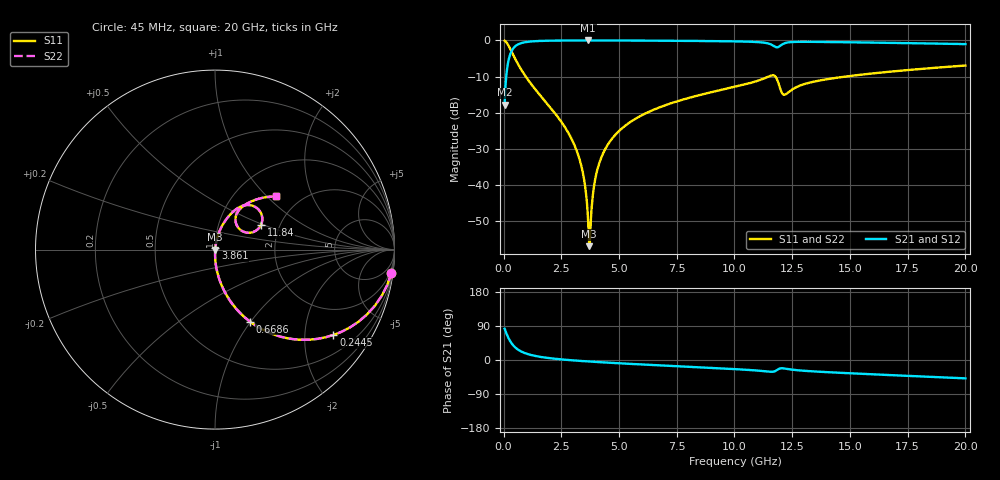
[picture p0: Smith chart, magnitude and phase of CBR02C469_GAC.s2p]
! S-parameter model data by Modelithics Inc.  support@modelithics.com 813-866-6335  Tampa FL USA
! S-Parameter data specifications:
! Substrate: 20-mil Rogers 4350B, substrate thickness, H=0.508mm, Dielectric constant, Er=3.75
! PCB Mounting Pad Footprint: Pad width, PadW=0.32mm , Pad length, PadL=0.37mm , Pad gap, PadG (edge-to-edge)=0.19mm , Reference planes=0.93mm apart
#  GHz  S  MA  R 50
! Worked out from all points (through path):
!   801 points, 45 MHz to 20 GHz, reference 50 ohm
!   highest |S21| = -0.01 dB at 3.662 GHz (marker M1); lowest = -17.7 dB at 45 MHz (marker M2)
!   group delay of S21, straight-line fit = 9.17 ps
!   lowest |S11| = -56.8 dB at 3.712 GHz (marker M3), VSWR 1.00, Z = 50.1 - j0.0492 ohm
!   |S11| at or under -10 dB: 961.4 MHz to 11.47 GHz (10.5 GHz wide, 169 % of centre); 11.77 GHz to 14.79 GHz (3.013 GHz wide, 22.7 % of centre)
!   |S22| runs from -56.8 to -0.1 dB; largest |S21 - S12| = 0
!   S11 on the Smith chart (normalised r, x): 45 MHz: 1, -15; 244.6 MHz: 0.99, -2.78; 668.6 MHz: 0.99, -0.99; 3.861 GHz: 1.00, +0.01; 11.84 GHz: 1.60, +0.48; 20 GHz: 1.52, +1.13
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0.045  0.9915 -7.5  0.1299 82.5  0.1299 82.5  0.9915 -7.5
0.24455  0.8133 -35.8  0.5814 54.2  0.5814 54.2  0.8133 -35.8
0.668594  0.445 -64.2  0.8946 25.7  0.8946 25.7  0.445 -64.2
1.292188  0.2276 -78.0  0.9727 11.8  0.9727 11.8  0.2276 -78.0
2.713981  0.05927 -88.3  0.9969 0.5  0.9969 0.5  0.05927 -88.3
3.387462  0.01744 -88.2  0.9984 -2.7  0.9984 -2.7  0.01744 -88.2
3.537125  0.009448 -85.0  0.9985 -3.3  0.9985 -3.3  0.009448 -85.0
3.661844  0.003222 -68.4  0.9985 -3.8  0.9985 -3.8  0.003222 -68.4
3.711731  0.001443 -19.9  0.9985 -4.0  0.9985 -4.0  0.001443 -19.9
3.786563  0.003598 62.9  0.9985 -4.3  0.9985 -4.3  0.003598 62.9
3.861394  0.007099 74.0  0.9985 -4.6  0.9985 -4.6  0.007099 74.0
4.110831  0.0187 80.1  0.9983 -5.5  0.9983 -5.5  0.0187 80.1
4.609706  0.04034 80.6  0.9976 -7.3  0.9976 -7.3  0.04034 80.6
5.43285  0.07258 78.7  0.9957 -10.0  0.9957 -10.0  0.07258 78.7
6.704981  0.1174 75.2  0.9913 -14.0  0.9913 -14.0  0.1174 75.2
10.0225  0.2291 65.0  0.9695 -24.1  0.9695 -24.1  0.2291 65.0
11.44429  0.3141 52.2  0.91 -30.5  0.91 -30.5  0.3141 52.2
11.84339  0.2899 28.0  0.803 -26.4  0.803 -26.4  0.2899 28.0
12.16766  0.178 43.0  0.9128 -22.5  0.9128 -22.5  0.178 43.0
13.36496  0.2663 58.4  0.9556 -29.9  0.9556 -29.9  0.2663 58.4
16.68248  0.3686 49.8  0.9259 -39.7  0.9259 -39.7  0.3686 49.8
20  0.4501 41.2  0.8895 -48.4  0.8895 -48.4  0.4501 41.2
